(* Logix 5000 AddOnInstructionDefinition export Banner_R90C_R95C_R130C_Param_v4; software revision 33.00; part 2 of 3 *)
(* tags used below, declared in another part *)
   Hub : Banner_Hub_v4;
   Port_Data : Banner_IOL_Port_v4;
   Port : INT;
   Type : INT;   // 4 = R90C-4B21, 8 = R95C-8B21, 22 = R95-8B22
   Control : DINT;
   Command_Being_Processed : BOOL;
   Update_Archive : BOOL;
   Index_Write_Inprocess : INT;
   Index_Write_Control : INT;
   Inprocess_Index : DINT;
   Index1 : SINT;
   Index6 : SINT;
   Index5 : SINT;
(* Banner_R90C_R95C_R130C_Param_v4, continued *)

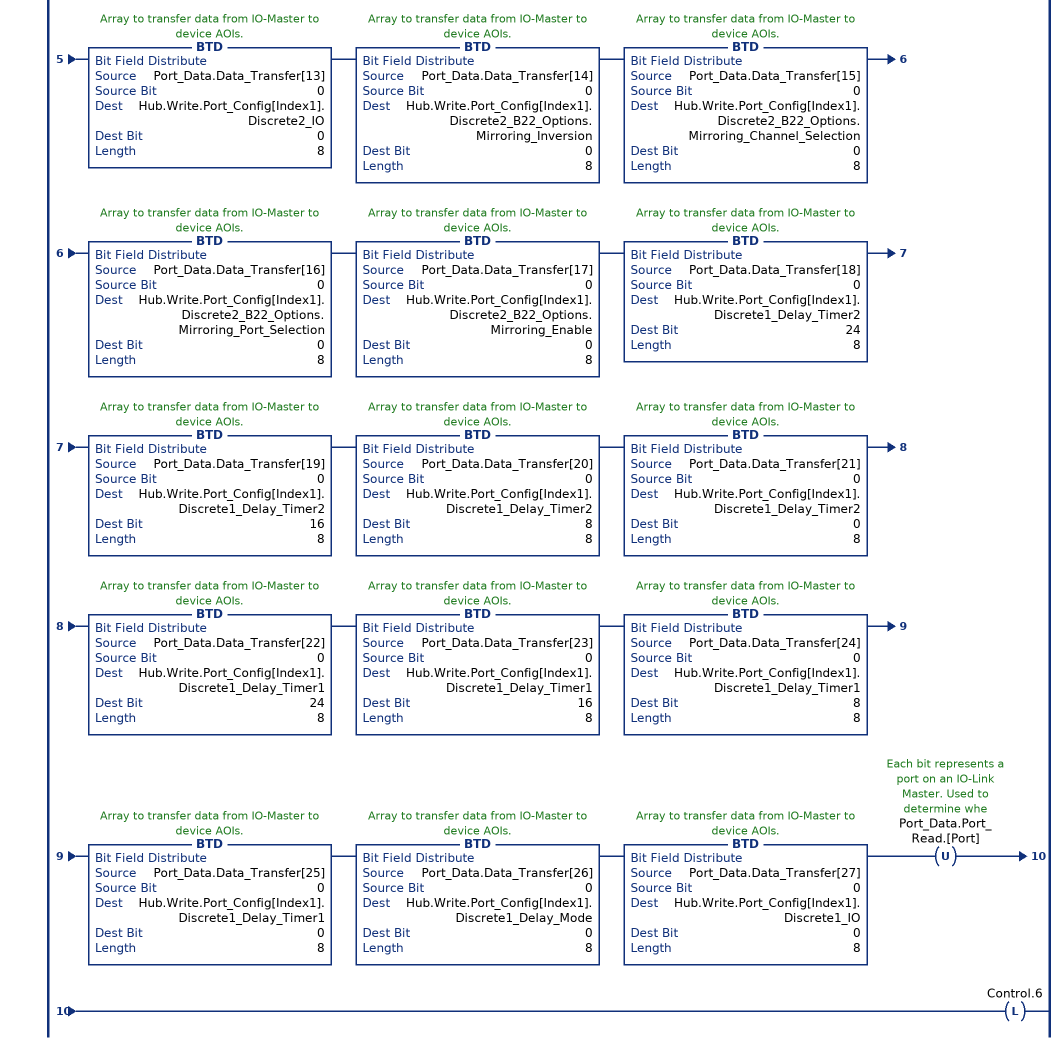
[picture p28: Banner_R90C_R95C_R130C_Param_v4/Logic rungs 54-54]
   54: XIC(Control.5)XIO(Control.6)GEQ(Hub.Command,13)LEQ(Hub.Command,20)EQU(Type,22)BTD(Port_Data.Data_Transfer[0],0,Hub.Write.Port_Config[Index1].Discrete2_B22_Options.Mirroring_Inversion,0,8)BTD(Port_Data.Data_Transfer[1],0,Hub.Write.Port_Config[Index1].Discrete2_B22_Options.Mirroring_Channel_Selection,0,8)BTD(Port_Data.Data_Transfer[2],0,Hub.Write.Port_Config[Index1].Discrete2_B22_Options.Mirroring_Port_Selection,0,8)BTD(Port_Data.Data_Transfer[3],0,Hub.Write.Port_Config[Index1].Discrete2_B22_Options.Mirroring_Enable,0,8)BTD(Port_Data.Data_Transfer[4],0,Hub.Write.Port_Config[Index1].Discrete2_Delay_Timer2,24,8)BTD(Port_Data.Data_Transfer[5],0,Hub.Write.Port_Config[Index1].Discrete2_Delay_Timer2,16,8)BTD(Port_Data.Data_Transfer[6],0,Hub.Write.Port_Config[Index1].Discrete2_Delay_Timer2,8,8)BTD(Port_Data.Data_Transfer[7],0,Hub.Write.Port_Config[Index1].Discrete2_Delay_Timer2,0,8)BTD(Port_Data.Data_Transfer[8],0,Hub.Write.Port_Config[Index1].Discrete2_Delay_Timer1,24,8)BTD(Port_Data.Data_Transfer[9],0,Hub.Write.Port_Config[Index1].Discrete2_Delay_Timer1,16,8)BTD(Port_Data.Data_Transfer[10],0,Hub.Write.Port_Config[Index1].Discrete2_Delay_Timer1,8,8)BTD(Port_Data.Data_Transfer[11],0,Hub.Write.Port_Config[Index1].Discrete2_Delay_Timer1,0,8)BTD(Port_Data.Data_Transfer[12],0,Hub.Write.Port_Config[Index1].Discrete2_Delay_Mode,0,8)BTD(Port_Data.Data_Transfer[13],0,Hub.Write.Port_Config[Index1].Discrete2_IO,0,8)BTD(Port_Data.Data_Transfer[14],0,Hub.Write.Port_Config[Index1].Discrete2_B22_Options.Mirroring_Inversion,0,8)BTD(Port_Data.Data_Transfer[15],0,Hub.Write.Port_Config[Index1].Discrete2_B22_Options.Mirroring_Channel_Selection,0,8)BTD(Port_Data.Data_Transfer[16],0,Hub.Write.Port_Config[Index1].Discrete2_B22_Options.Mirroring_Port_Selection,0,8)BTD(Port_Data.Data_Transfer[17],0,Hub.Write.Port_Config[Index1].Discrete2_B22_Options.Mirroring_Enable,0,8)BTD(Port_Data.Data_Transfer[18],0,Hub.Write.Port_Config[Index1].Discrete1_Delay_Timer2,24,8)BTD(Port_Data.Data_Transfer[19],0,Hub.Write.Port_Config[Index1].Discrete1_Delay_Timer2,16,8)BTD(Port_Data.Data_Transfer[20],0,Hub.Write.Port_Config[Index1].Discrete1_Delay_Timer2,8,8)BTD(Port_Data.Data_Transfer[21],0,Hub.Write.Port_Config[Index1].Discrete1_Delay_Timer2,0,8)BTD(Port_Data.Data_Transfer[22],0,Hub.Write.Port_Config[Index1].Discrete1_Delay_Timer1,24,8)BTD(Port_Data.Data_Transfer[23],0,Hub.Write.Port_Config[Index1].Discrete1_Delay_Timer1,16,8)BTD(Port_Data.Data_Transfer[24],0,Hub.Write.Port_Config[Index1].Discrete1_Delay_Timer1,8,8)BTD(Port_Data.Data_Transfer[25],0,Hub.Write.Port_Config[Index1].Discrete1_Delay_Timer1,0,8)BTD(Port_Data.Data_Transfer[26],0,Hub.Write.Port_Config[Index1].Discrete1_Delay_Mode,0,8)BTD(Port_Data.Data_Transfer[27],0,Hub.Write.Port_Config[Index1].Discrete1_IO,0,8)OTU(Port_Data.Port_Read.[Port])OTL(Control.6);
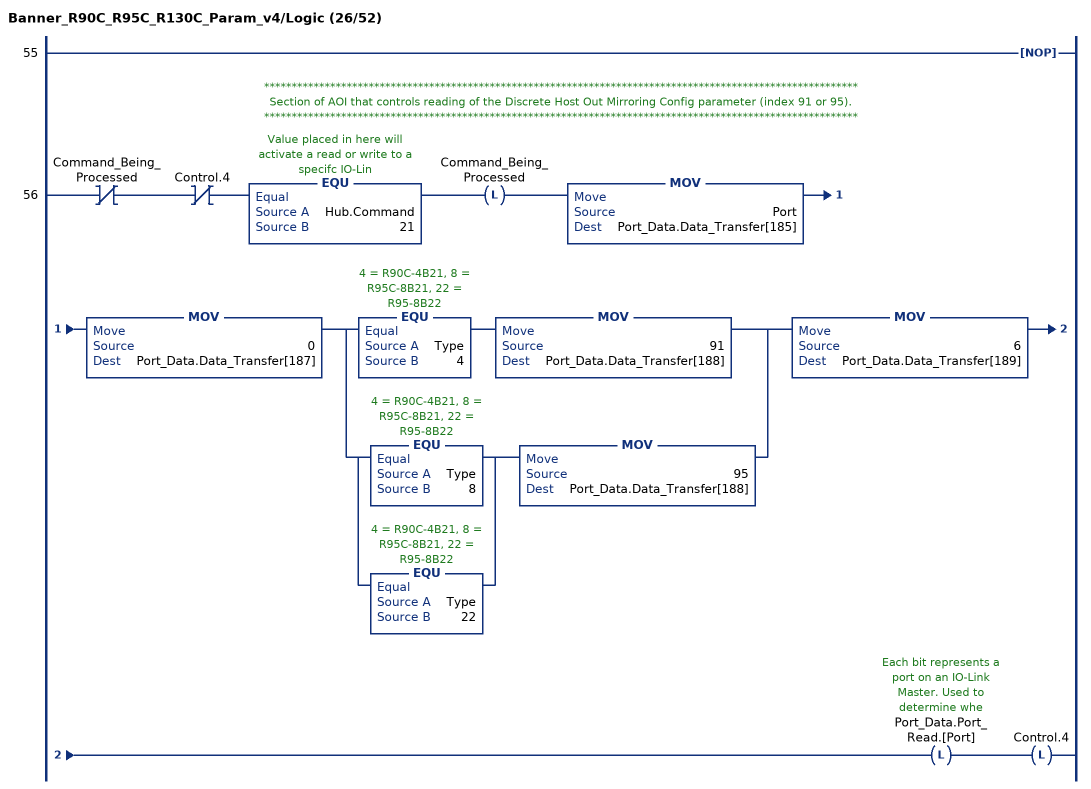
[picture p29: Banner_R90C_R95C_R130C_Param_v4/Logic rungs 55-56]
   55: NOP();
   // ************************************************************************************************************
   // Section of AOI that controls reading of the Discrete Host Out Mirroring Config parameter (index 91 or 95).
   // ************************************************************************************************************
   56: XIO(Command_Being_Processed)XIO(Control.4)EQU(Hub.Command,21)OTL(Command_Being_Processed)MOV(Port,Port_Data.Data_Transfer[185])MOV(0,Port_Data.Data_Transfer[187])[EQU(Type,4) MOV(91,Port_Data.Data_Transfer[188]) ,[EQU(Type,8) ,EQU(Type,22) ] MOV(95,Port_Data.Data_Transfer[188]) ]MOV(6,Port_Data.Data_Transfer[189])OTL(Port_Data.Port_Read.[Port])OTL(Control.4);
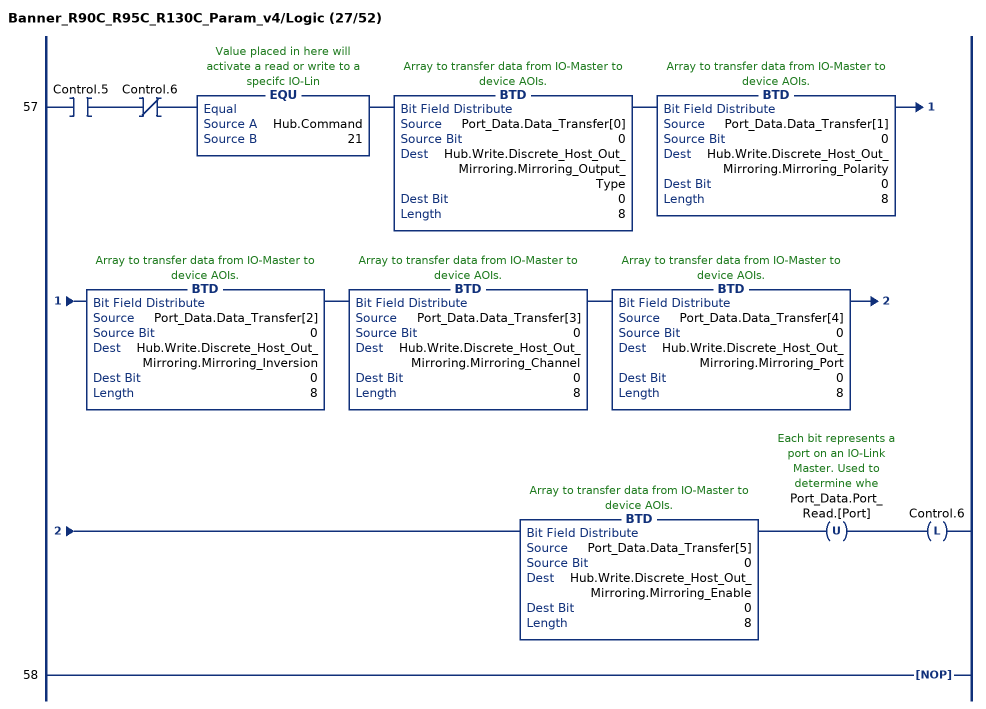
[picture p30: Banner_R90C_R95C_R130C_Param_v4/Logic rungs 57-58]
   57: XIC(Control.5)XIO(Control.6)EQU(Hub.Command,21)BTD(Port_Data.Data_Transfer[0],0,Hub.Write.Discrete_Host_Out_Mirroring.Mirroring_Output_Type,0,8)BTD(Port_Data.Data_Transfer[1],0,Hub.Write.Discrete_Host_Out_Mirroring.Mirroring_Polarity,0,8)BTD(Port_Data.Data_Transfer[2],0,Hub.Write.Discrete_Host_Out_Mirroring.Mirroring_Inversion,0,8)BTD(Port_Data.Data_Transfer[3],0,Hub.Write.Discrete_Host_Out_Mirroring.Mirroring_Channel,0,8)BTD(Port_Data.Data_Transfer[4],0,Hub.Write.Discrete_Host_Out_Mirroring.Mirroring_Port,0,8)BTD(Port_Data.Data_Transfer[5],0,Hub.Write.Discrete_Host_Out_Mirroring.Mirroring_Enable,0,8)OTU(Port_Data.Port_Read.[Port])OTL(Control.6);
   58: NOP();
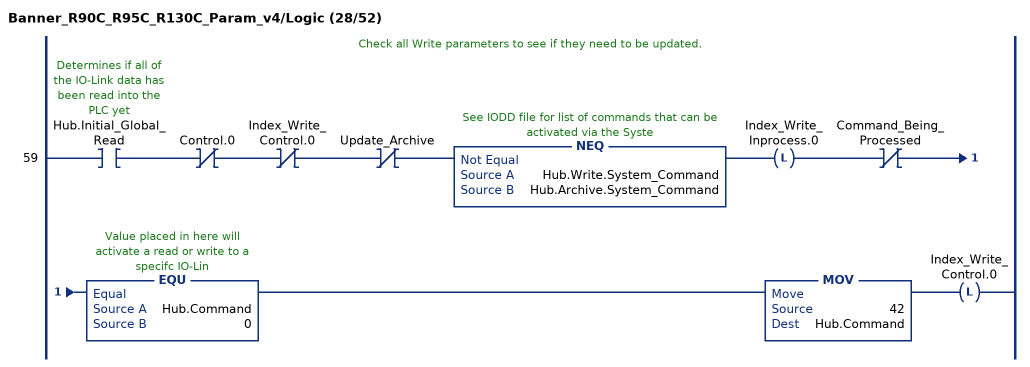
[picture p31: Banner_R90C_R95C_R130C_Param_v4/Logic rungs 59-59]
   // Check all Write parameters to see if they need to be updated.
   59: XIC(Hub.Initial_Global_Read)XIO(Control.0)XIO(Index_Write_Control.0)XIO(Update_Archive)NEQ(Hub.Write.System_Command,Hub.Archive.System_Command)OTL(Index_Write_Inprocess.0)XIO(Command_Being_Processed)EQU(Hub.Command,0)MOV(42,Hub.Command)OTL(Index_Write_Control.0);
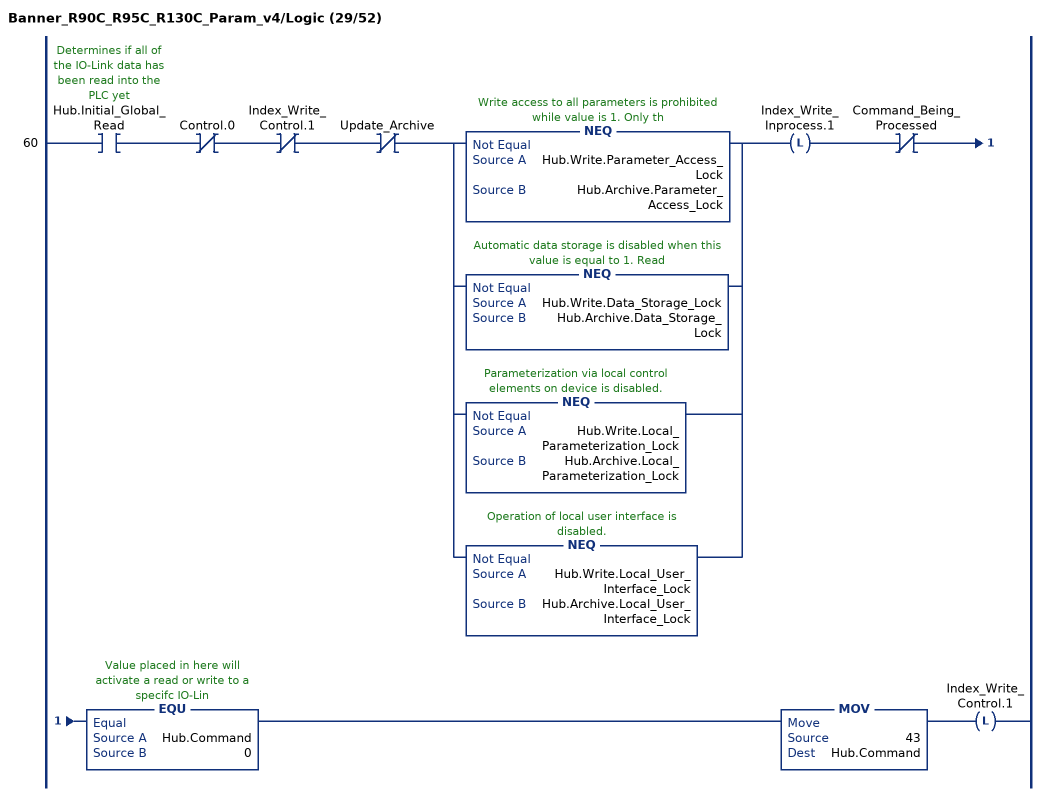
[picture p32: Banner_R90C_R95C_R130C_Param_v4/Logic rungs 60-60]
   60: XIC(Hub.Initial_Global_Read)XIO(Control.0)XIO(Index_Write_Control.1)XIO(Update_Archive)[NEQ(Hub.Write.Parameter_Access_Lock,Hub.Archive.Parameter_Access_Lock) ,NEQ(Hub.Write.Data_Storage_Lock,Hub.Archive.Data_Storage_Lock) ,NEQ(Hub.Write.Local_Parameterization_Lock,Hub.Archive.Local_Parameterization_Lock) ,NEQ(Hub.Write.Local_User_Interface_Lock,Hub.Archive.Local_User_Interface_Lock) ]OTL(Index_Write_Inprocess.1)XIO(Command_Being_Processed)EQU(Hub.Command,0)MOV(43,Hub.Command)OTL(Index_Write_Control.1);
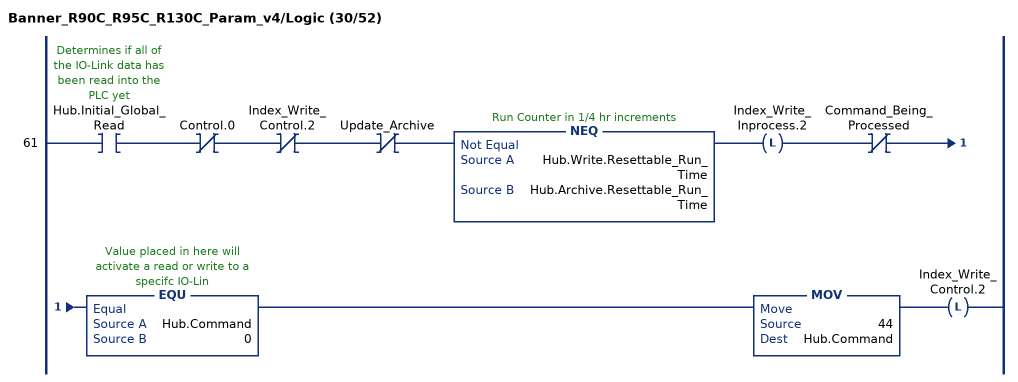
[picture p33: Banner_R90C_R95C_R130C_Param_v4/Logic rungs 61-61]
   61: XIC(Hub.Initial_Global_Read)XIO(Control.0)XIO(Index_Write_Control.2)XIO(Update_Archive)NEQ(Hub.Write.Resettable_Run_Time,Hub.Archive.Resettable_Run_Time)OTL(Index_Write_Inprocess.2)XIO(Command_Being_Processed)EQU(Hub.Command,0)MOV(44,Hub.Command)OTL(Index_Write_Control.2);
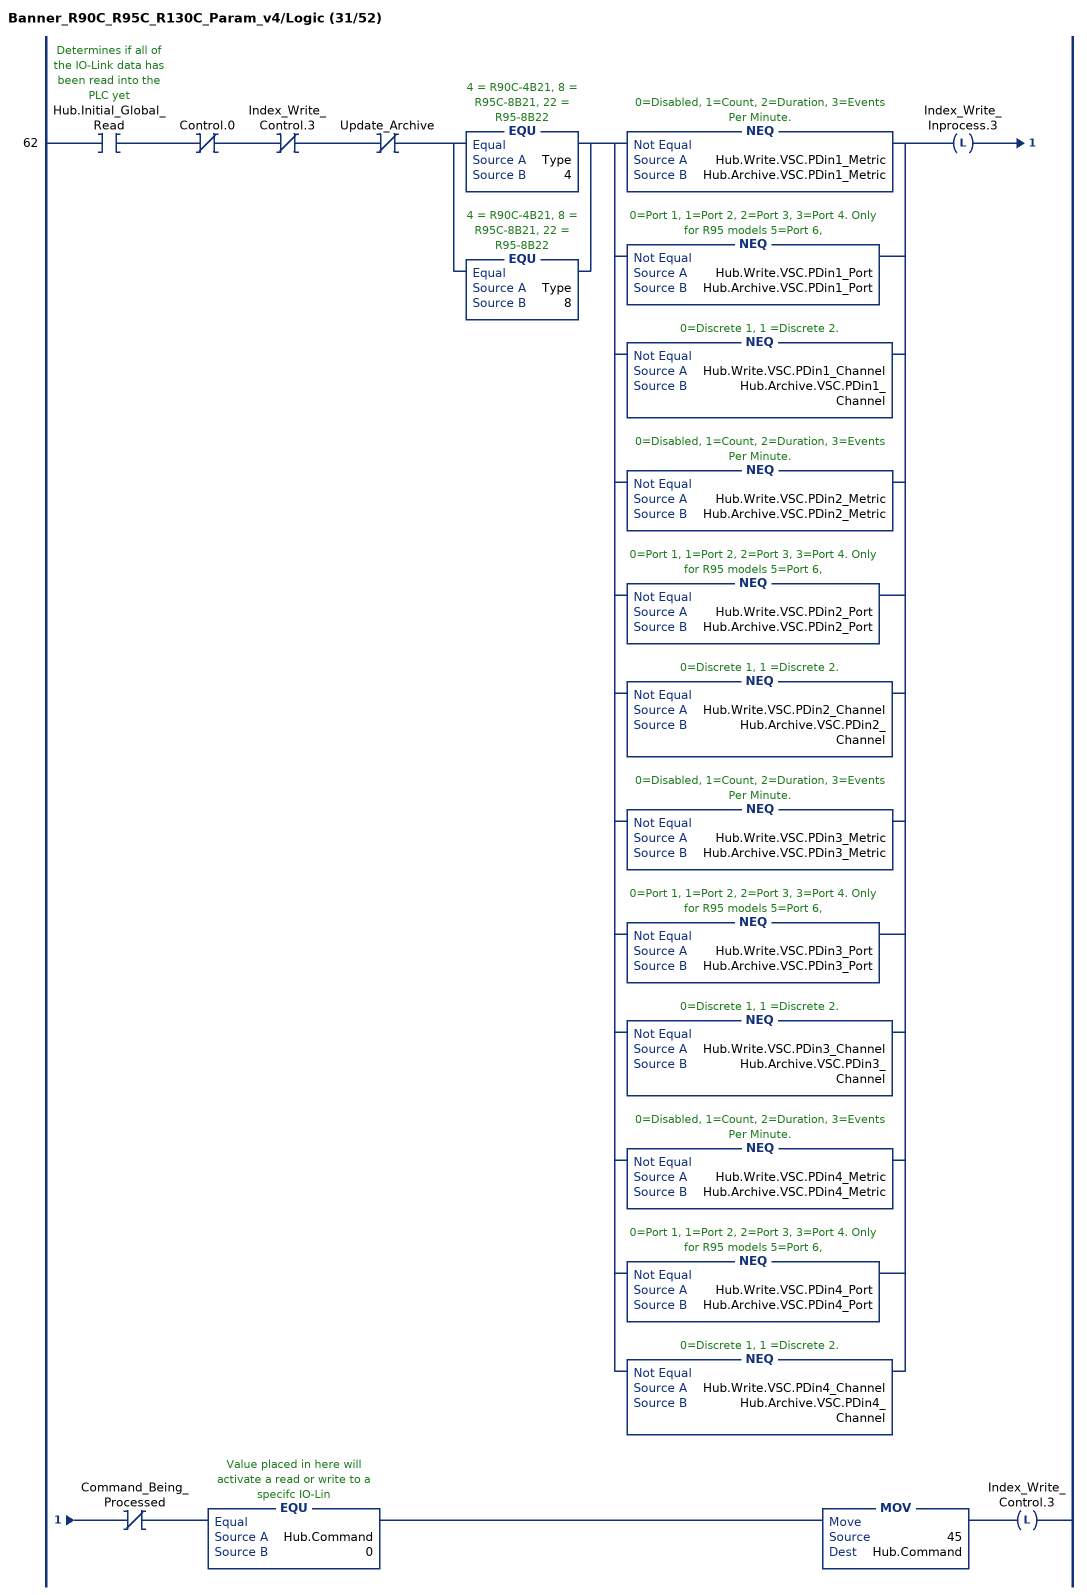
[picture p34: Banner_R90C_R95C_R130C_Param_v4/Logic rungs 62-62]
   62: XIC(Hub.Initial_Global_Read)XIO(Control.0)XIO(Index_Write_Control.3)XIO(Update_Archive)[EQU(Type,4) ,EQU(Type,8) ][NEQ(Hub.Write.VSC.PDin1_Metric,Hub.Archive.VSC.PDin1_Metric) ,NEQ(Hub.Write.VSC.PDin1_Port,Hub.Archive.VSC.PDin1_Port) ,NEQ(Hub.Write.VSC.PDin1_Channel,Hub.Archive.VSC.PDin1_Channel) ,NEQ(Hub.Write.VSC.PDin2_Metric,Hub.Archive.VSC.PDin2_Metric) ,NEQ(Hub.Write.VSC.PDin2_Port,Hub.Archive.VSC.PDin2_Port) ,NEQ(Hub.Write.VSC.PDin2_Channel,Hub.Archive.VSC.PDin2_Channel) ,NEQ(Hub.Write.VSC.PDin3_Metric,Hub.Archive.VSC.PDin3_Metric) ,NEQ(Hub.Write.VSC.PDin3_Port,Hub.Archive.VSC.PDin3_Port) ,NEQ(Hub.Write.VSC.PDin3_Channel,Hub.Archive.VSC.PDin3_Channel) ,NEQ(Hub.Write.VSC.PDin4_Metric,Hub.Archive.VSC.PDin4_Metric) ,NEQ(Hub.Write.VSC.PDin4_Port,Hub.Archive.VSC.PDin4_Port) ,NEQ(Hub.Write.VSC.PDin4_Channel,Hub.Archive.VSC.PDin4_Channel) ]OTL(Index_Write_Inprocess.3)XIO(Command_Being_Processed)EQU(Hub.Command,0)MOV(45,Hub.Command)OTL(Index_Write_Control.3);
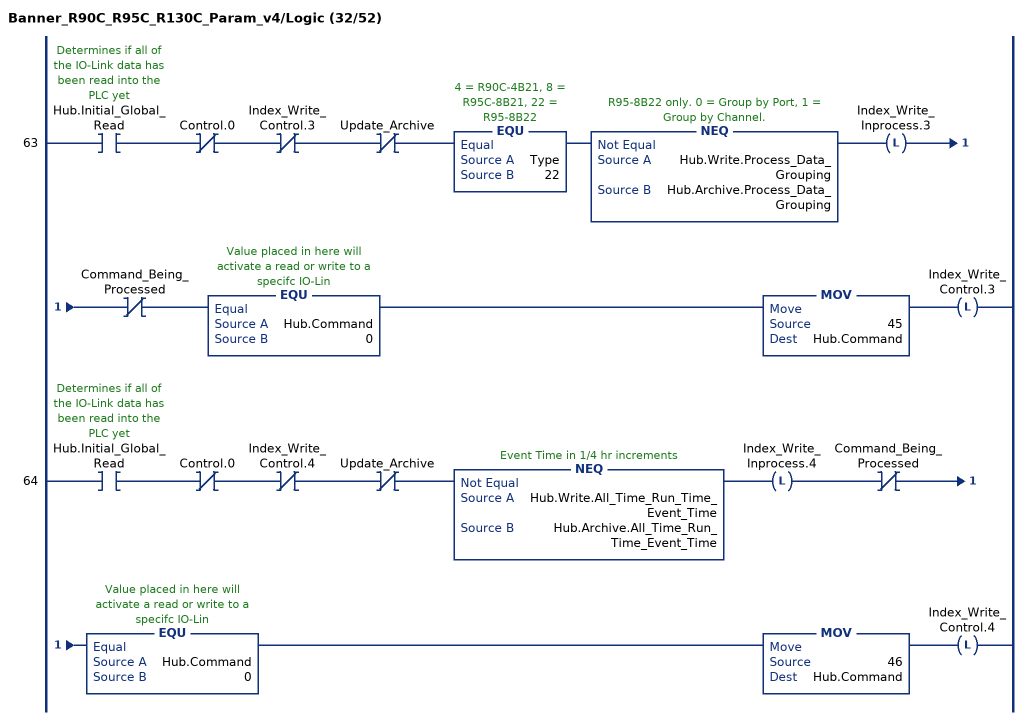
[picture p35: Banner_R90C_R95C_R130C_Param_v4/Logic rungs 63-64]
   63: XIC(Hub.Initial_Global_Read)XIO(Control.0)XIO(Index_Write_Control.3)XIO(Update_Archive)EQU(Type,22)NEQ(Hub.Write.Process_Data_Grouping,Hub.Archive.Process_Data_Grouping)OTL(Index_Write_Inprocess.3)XIO(Command_Being_Processed)EQU(Hub.Command,0)MOV(45,Hub.Command)OTL(Index_Write_Control.3);
   64: XIC(Hub.Initial_Global_Read)XIO(Control.0)XIO(Index_Write_Control.4)XIO(Update_Archive)NEQ(Hub.Write.All_Time_Run_Time_Event_Time,Hub.Archive.All_Time_Run_Time_Event_Time)OTL(Index_Write_Inprocess.4)XIO(Command_Being_Processed)EQU(Hub.Command,0)MOV(46,Hub.Command)OTL(Index_Write_Control.4);
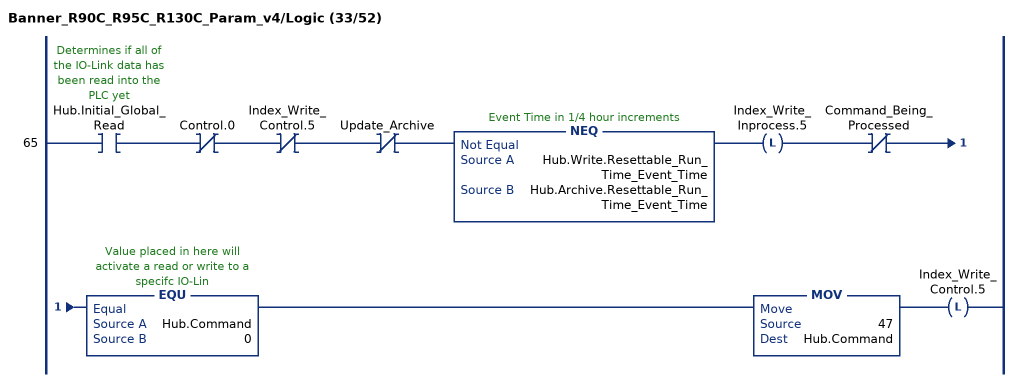
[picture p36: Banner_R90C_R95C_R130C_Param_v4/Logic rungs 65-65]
   65: XIC(Hub.Initial_Global_Read)XIO(Control.0)XIO(Index_Write_Control.5)XIO(Update_Archive)NEQ(Hub.Write.Resettable_Run_Time_Event_Time,Hub.Archive.Resettable_Run_Time_Event_Time)OTL(Index_Write_Inprocess.5)XIO(Command_Being_Processed)EQU(Hub.Command,0)MOV(47,Hub.Command)OTL(Index_Write_Control.5);
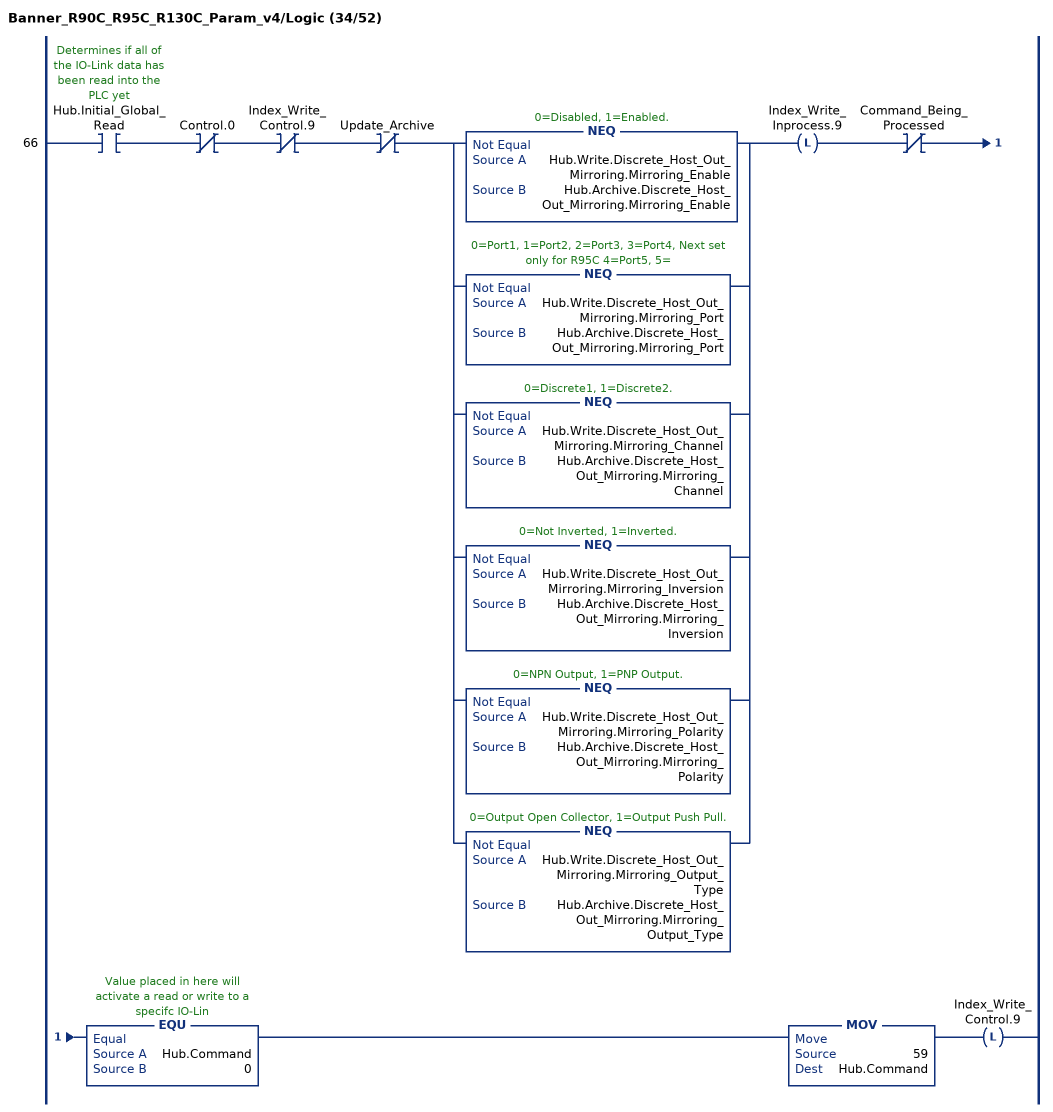
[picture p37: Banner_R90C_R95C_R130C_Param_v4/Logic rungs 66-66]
   66: XIC(Hub.Initial_Global_Read)XIO(Control.0)XIO(Index_Write_Control.9)XIO(Update_Archive)[NEQ(Hub.Write.Discrete_Host_Out_Mirroring.Mirroring_Enable,Hub.Archive.Discrete_Host_Out_Mirroring.Mirroring_Enable) ,NEQ(Hub.Write.Discrete_Host_Out_Mirroring.Mirroring_Port,Hub.Archive.Discrete_Host_Out_Mirroring.Mirroring_Port) ,NEQ(Hub.Write.Discrete_Host_Out_Mirroring.Mirroring_Channel,Hub.Archive.Discrete_Host_Out_Mirroring.Mirroring_Channel) ,NEQ(Hub.Write.Discrete_Host_Out_Mirroring.Mirroring_Inversion,Hub.Archive.Discrete_Host_Out_Mirroring.Mirroring_Inversion) ,NEQ(Hub.Write.Discrete_Host_Out_Mirroring.Mirroring_Polarity,Hub.Archive.Discrete_Host_Out_Mirroring.Mirroring_Polarity) ,NEQ(Hub.Write.Discrete_Host_Out_Mirroring.Mirroring_Output_Type,Hub.Archive.Discrete_Host_Out_Mirroring.Mirroring_Output_Type) ]OTL(Index_Write_Inprocess.9)XIO(Command_Being_Processed)EQU(Hub.Command,0)MOV(59,Hub.Command)OTL(Index_Write_Control.9);
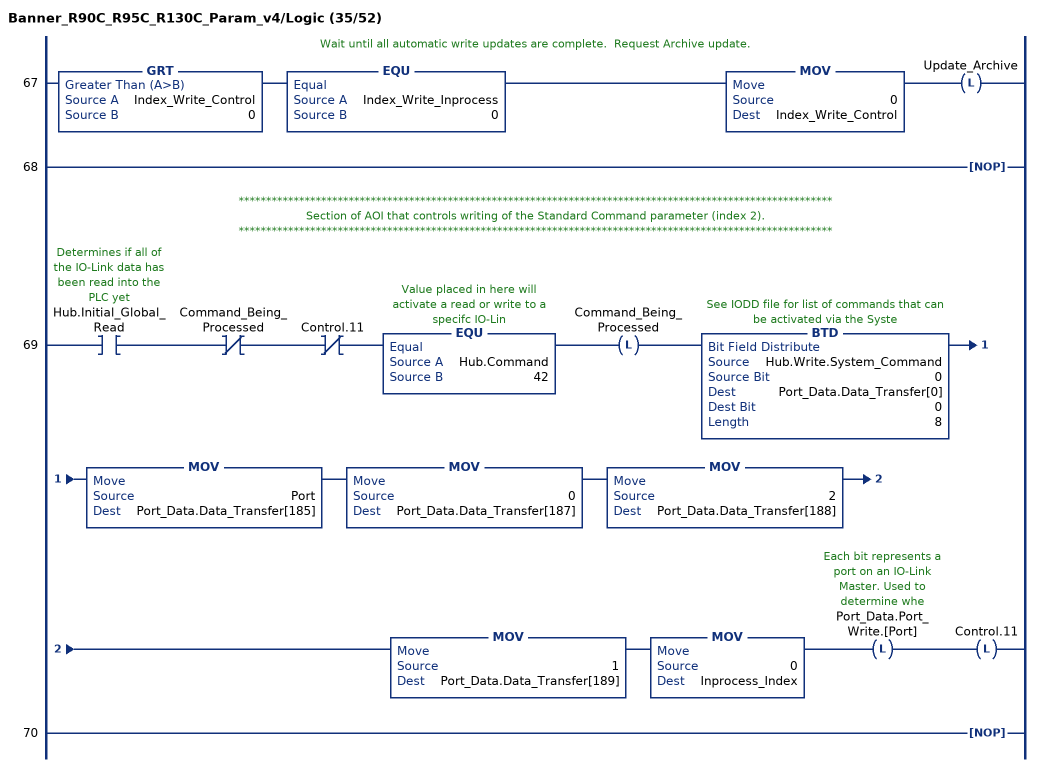
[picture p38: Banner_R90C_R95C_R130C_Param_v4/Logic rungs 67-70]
   // Wait until all automatic write updates are complete.  Request Archive update.
   67: GRT(Index_Write_Control,0)EQU(Index_Write_Inprocess,0)MOV(0,Index_Write_Control)OTL(Update_Archive);
   68: NOP();
   // ************************************************************************************************************
   // Section of AOI that controls writing of the Standard Command parameter (index 2).
   // ************************************************************************************************************
   69: XIC(Hub.Initial_Global_Read)XIO(Command_Being_Processed)XIO(Control.11)EQU(Hub.Command,42)OTL(Command_Being_Processed)BTD(Hub.Write.System_Command,0,Port_Data.Data_Transfer[0],0,8)MOV(Port,Port_Data.Data_Transfer[185])MOV(0,Port_Data.Data_Transfer[187])MOV(2,Port_Data.Data_Transfer[188])MOV(1,Port_Data.Data_Transfer[189])MOV(0,Inprocess_Index)OTL(Port_Data.Port_Write.[Port])OTL(Control.11);
   70: NOP();
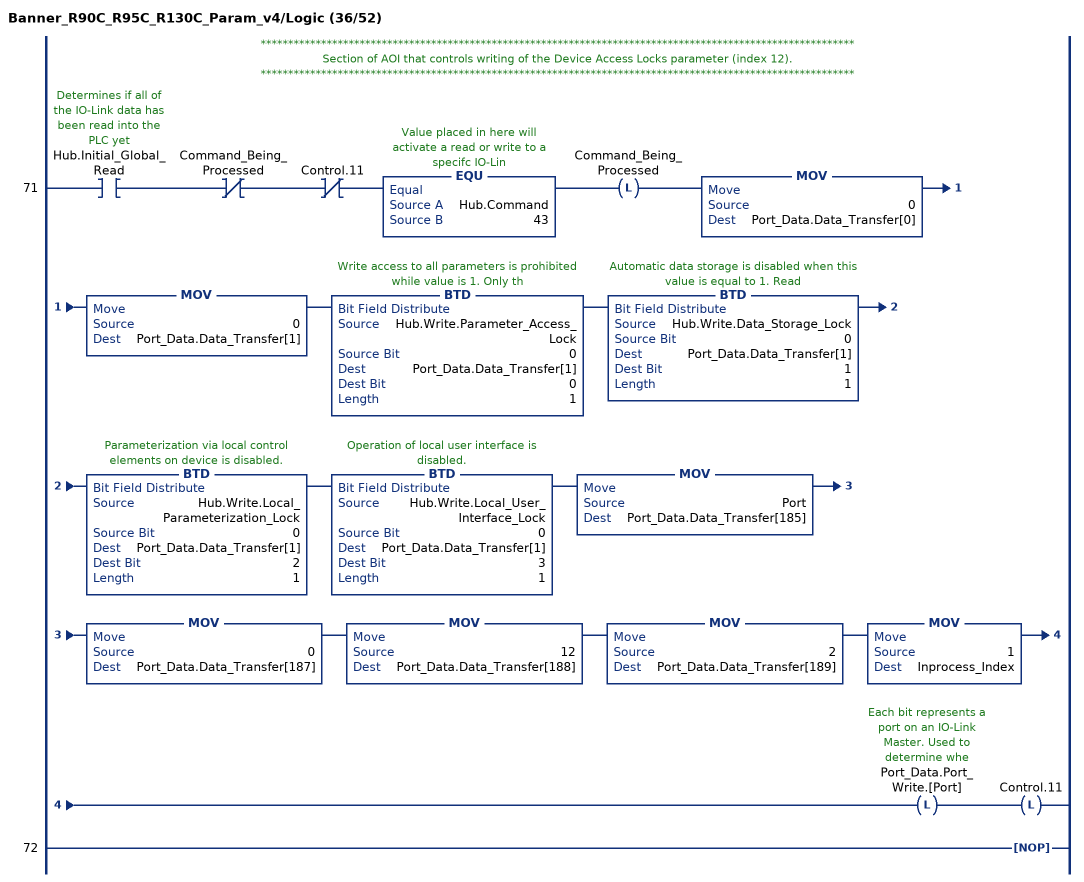
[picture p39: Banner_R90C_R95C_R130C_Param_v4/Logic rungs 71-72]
   // ************************************************************************************************************
   // Section of AOI that controls writing of the Device Access Locks parameter (index 12).
   // ************************************************************************************************************
   71: XIC(Hub.Initial_Global_Read)XIO(Command_Being_Processed)XIO(Control.11)EQU(Hub.Command,43)OTL(Command_Being_Processed)MOV(0,Port_Data.Data_Transfer[0])MOV(0,Port_Data.Data_Transfer[1])BTD(Hub.Write.Parameter_Access_Lock,0,Port_Data.Data_Transfer[1],0,1)BTD(Hub.Write.Data_Storage_Lock,0,Port_Data.Data_Transfer[1],1,1)BTD(Hub.Write.Local_Parameterization_Lock,0,Port_Data.Data_Transfer[1],2,1)BTD(Hub.Write.Local_User_Interface_Lock,0,Port_Data.Data_Transfer[1],3,1)MOV(Port,Port_Data.Data_Transfer[185])MOV(0,Port_Data.Data_Transfer[187])MOV(12,Port_Data.Data_Transfer[188])MOV(2,Port_Data.Data_Transfer[189])MOV(1,Inprocess_Index)OTL(Port_Data.Port_Write.[Port])OTL(Control.11);
   72: NOP();
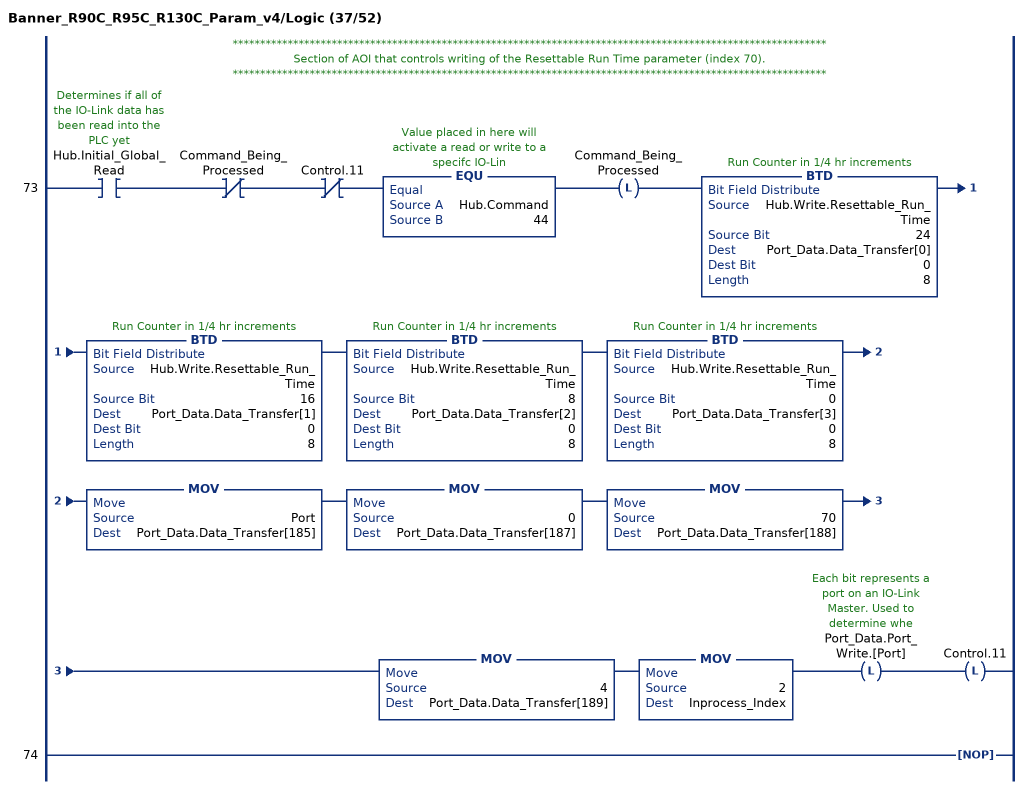
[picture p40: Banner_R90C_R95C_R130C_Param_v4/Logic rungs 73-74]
   // ************************************************************************************************************
   // Section of AOI that controls writing of the Resettable Run Time parameter (index 70).
   // ************************************************************************************************************
   73: XIC(Hub.Initial_Global_Read)XIO(Command_Being_Processed)XIO(Control.11)EQU(Hub.Command,44)OTL(Command_Being_Processed)BTD(Hub.Write.Resettable_Run_Time,24,Port_Data.Data_Transfer[0],0,8)BTD(Hub.Write.Resettable_Run_Time,16,Port_Data.Data_Transfer[1],0,8)BTD(Hub.Write.Resettable_Run_Time,8,Port_Data.Data_Transfer[2],0,8)BTD(Hub.Write.Resettable_Run_Time,0,Port_Data.Data_Transfer[3],0,8)MOV(Port,Port_Data.Data_Transfer[185])MOV(0,Port_Data.Data_Transfer[187])MOV(70,Port_Data.Data_Transfer[188])MOV(4,Port_Data.Data_Transfer[189])MOV(2,Inprocess_Index)OTL(Port_Data.Port_Write.[Port])OTL(Control.11);
   74: NOP();
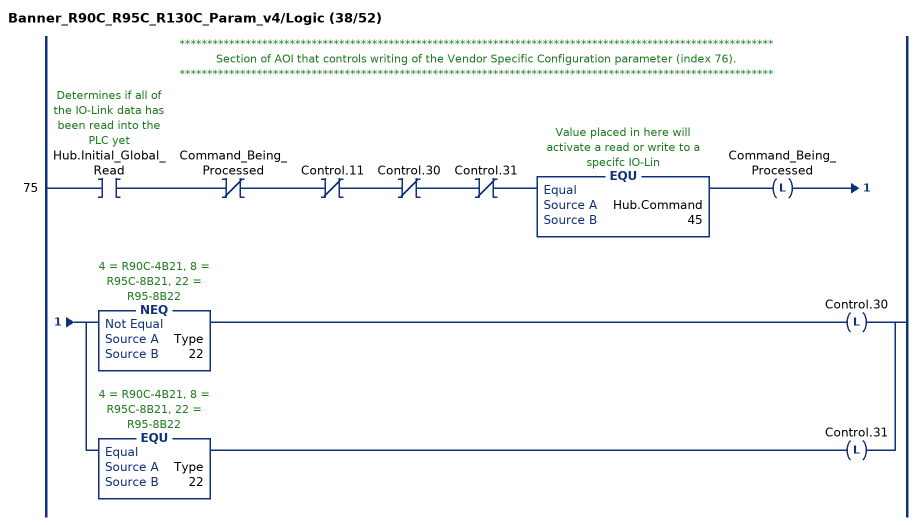
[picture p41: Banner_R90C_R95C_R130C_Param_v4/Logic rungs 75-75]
   // ************************************************************************************************************
   // Section of AOI that controls writing of the Vendor Specific Configuration parameter (index 76).
   // ************************************************************************************************************
   75: XIC(Hub.Initial_Global_Read)XIO(Command_Being_Processed)XIO(Control.11)XIO(Control.30)XIO(Control.31)EQU(Hub.Command,45)OTL(Command_Being_Processed)[NEQ(Type,22) OTL(Control.30) ,EQU(Type,22) OTL(Control.31) ];
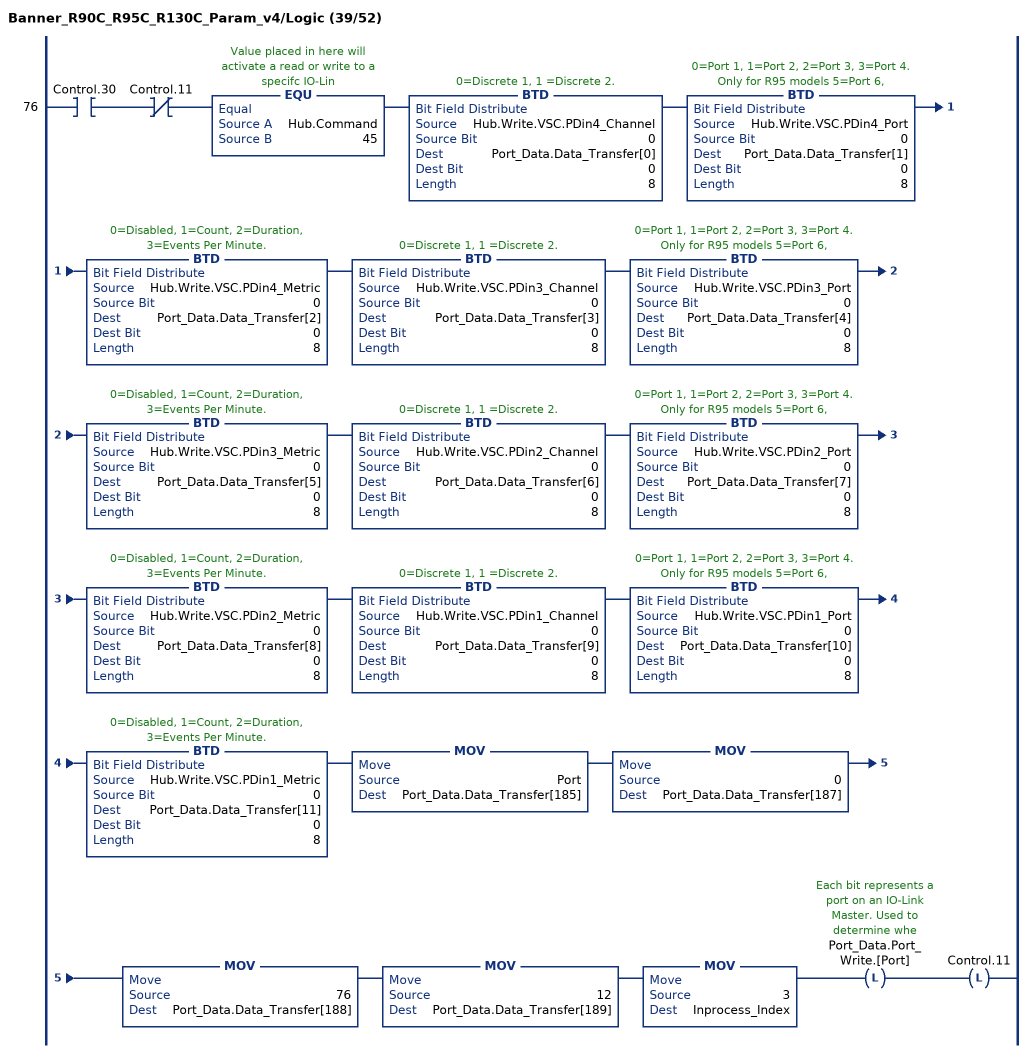
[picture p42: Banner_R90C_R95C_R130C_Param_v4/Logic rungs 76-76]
   76: XIC(Control.30)XIO(Control.11)EQU(Hub.Command,45)BTD(Hub.Write.VSC.PDin4_Channel,0,Port_Data.Data_Transfer[0],0,8)BTD(Hub.Write.VSC.PDin4_Port,0,Port_Data.Data_Transfer[1],0,8)BTD(Hub.Write.VSC.PDin4_Metric,0,Port_Data.Data_Transfer[2],0,8)BTD(Hub.Write.VSC.PDin3_Channel,0,Port_Data.Data_Transfer[3],0,8)BTD(Hub.Write.VSC.PDin3_Port,0,Port_Data.Data_Transfer[4],0,8)BTD(Hub.Write.VSC.PDin3_Metric,0,Port_Data.Data_Transfer[5],0,8)BTD(Hub.Write.VSC.PDin2_Channel,0,Port_Data.Data_Transfer[6],0,8)BTD(Hub.Write.VSC.PDin2_Port,0,Port_Data.Data_Transfer[7],0,8)BTD(Hub.Write.VSC.PDin2_Metric,0,Port_Data.Data_Transfer[8],0,8)BTD(Hub.Write.VSC.PDin1_Channel,0,Port_Data.Data_Transfer[9],0,8)BTD(Hub.Write.VSC.PDin1_Port,0,Port_Data.Data_Transfer[10],0,8)BTD(Hub.Write.VSC.PDin1_Metric,0,Port_Data.Data_Transfer[11],0,8)MOV(Port,Port_Data.Data_Transfer[185])MOV(0,Port_Data.Data_Transfer[187])MOV(76,Port_Data.Data_Transfer[188])MOV(12,Port_Data.Data_Transfer[189])MOV(3,Inprocess_Index)OTL(Port_Data.Port_Write.[Port])OTL(Control.11);
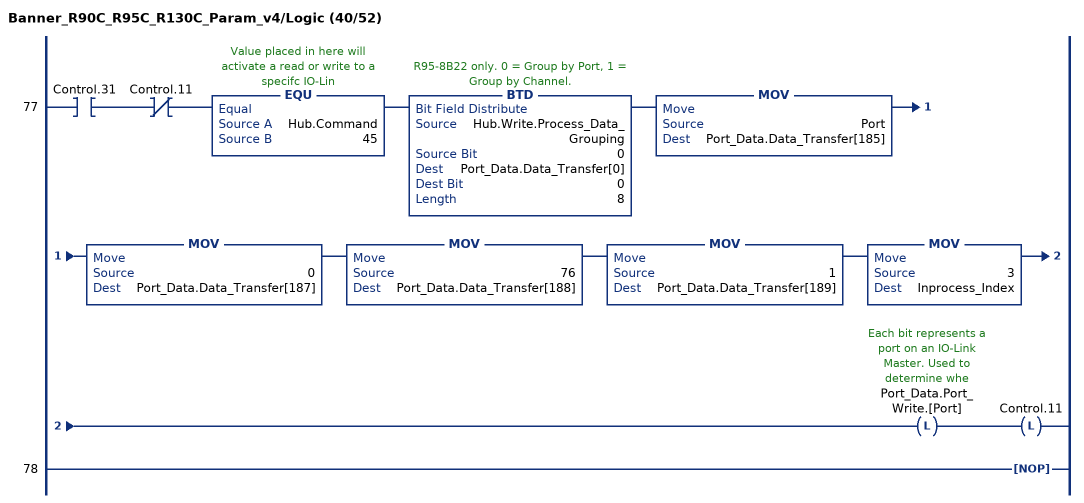
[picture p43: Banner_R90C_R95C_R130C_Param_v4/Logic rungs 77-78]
   77: XIC(Control.31)XIO(Control.11)EQU(Hub.Command,45)BTD(Hub.Write.Process_Data_Grouping,0,Port_Data.Data_Transfer[0],0,8)MOV(Port,Port_Data.Data_Transfer[185])MOV(0,Port_Data.Data_Transfer[187])MOV(76,Port_Data.Data_Transfer[188])MOV(1,Port_Data.Data_Transfer[189])MOV(3,Inprocess_Index)OTL(Port_Data.Port_Write.[Port])OTL(Control.11);
   78: NOP();
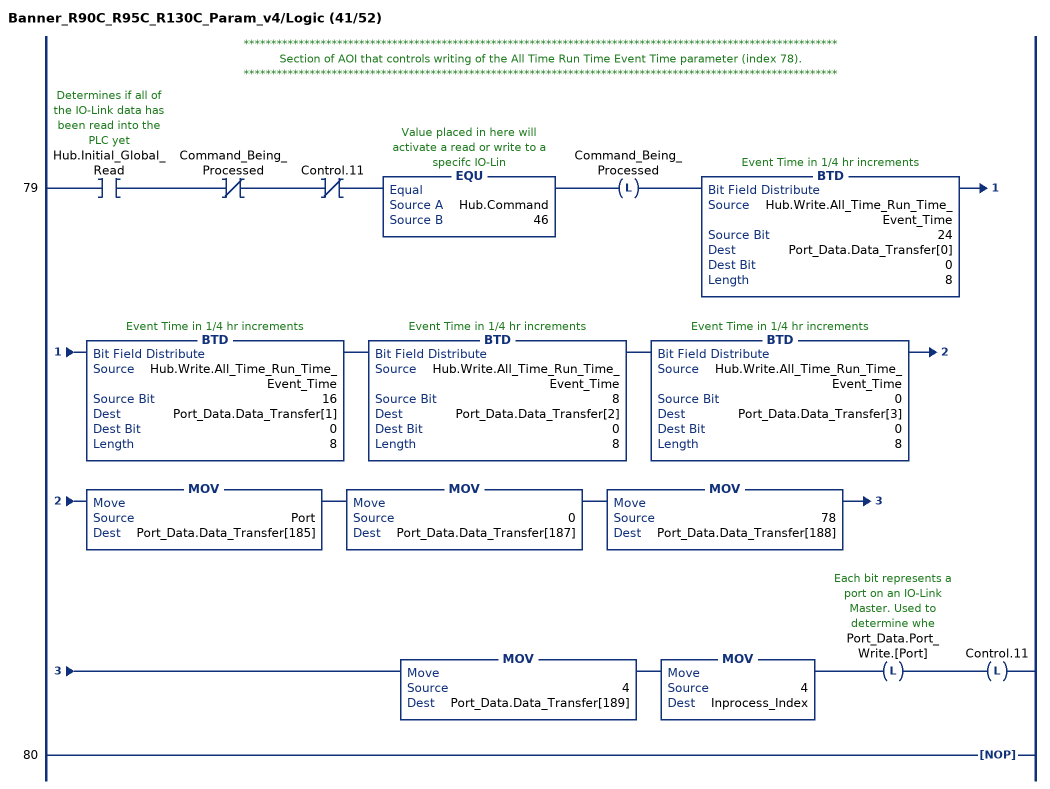
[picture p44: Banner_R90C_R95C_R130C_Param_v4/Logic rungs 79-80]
   // ************************************************************************************************************
   // Section of AOI that controls writing of the All Time Run Time Event Time parameter (index 78).
   // ************************************************************************************************************
   79: XIC(Hub.Initial_Global_Read)XIO(Command_Being_Processed)XIO(Control.11)EQU(Hub.Command,46)OTL(Command_Being_Processed)BTD(Hub.Write.All_Time_Run_Time_Event_Time,24,Port_Data.Data_Transfer[0],0,8)BTD(Hub.Write.All_Time_Run_Time_Event_Time,16,Port_Data.Data_Transfer[1],0,8)BTD(Hub.Write.All_Time_Run_Time_Event_Time,8,Port_Data.Data_Transfer[2],0,8)BTD(Hub.Write.All_Time_Run_Time_Event_Time,0,Port_Data.Data_Transfer[3],0,8)MOV(Port,Port_Data.Data_Transfer[185])MOV(0,Port_Data.Data_Transfer[187])MOV(78,Port_Data.Data_Transfer[188])MOV(4,Port_Data.Data_Transfer[189])MOV(4,Inprocess_Index)OTL(Port_Data.Port_Write.[Port])OTL(Control.11);
   80: NOP();
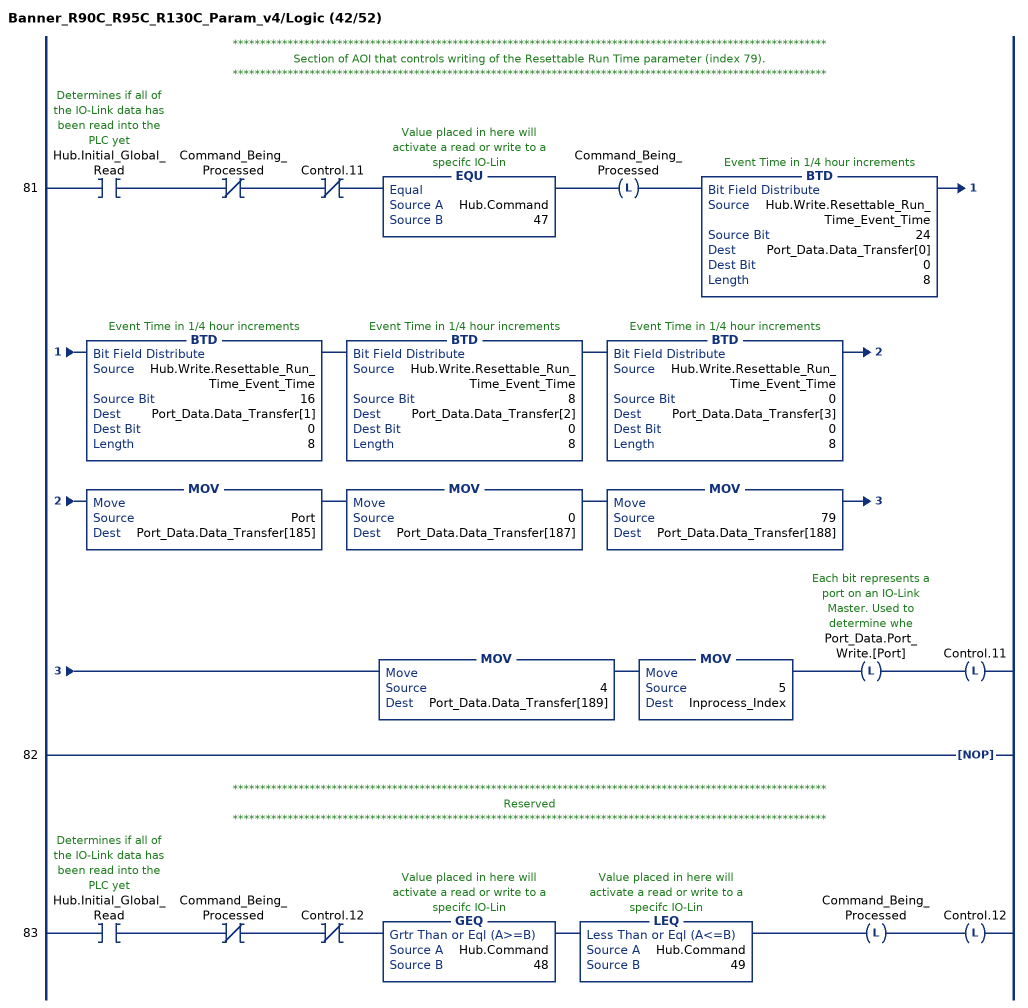
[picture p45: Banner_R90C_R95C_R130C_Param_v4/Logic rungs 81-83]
   // ************************************************************************************************************
   // Section of AOI that controls writing of the Resettable Run Time parameter (index 79).
   // ************************************************************************************************************
   81: XIC(Hub.Initial_Global_Read)XIO(Command_Being_Processed)XIO(Control.11)EQU(Hub.Command,47)OTL(Command_Being_Processed)BTD(Hub.Write.Resettable_Run_Time_Event_Time,24,Port_Data.Data_Transfer[0],0,8)BTD(Hub.Write.Resettable_Run_Time_Event_Time,16,Port_Data.Data_Transfer[1],0,8)BTD(Hub.Write.Resettable_Run_Time_Event_Time,8,Port_Data.Data_Transfer[2],0,8)BTD(Hub.Write.Resettable_Run_Time_Event_Time,0,Port_Data.Data_Transfer[3],0,8)MOV(Port,Port_Data.Data_Transfer[185])MOV(0,Port_Data.Data_Transfer[187])MOV(79,Port_Data.Data_Transfer[188])MOV(4,Port_Data.Data_Transfer[189])MOV(5,Inprocess_Index)OTL(Port_Data.Port_Write.[Port])OTL(Control.11);
   82: NOP();
   // ************************************************************************************************************
   // Reserved
   // ************************************************************************************************************
   83: XIC(Hub.Initial_Global_Read)XIO(Command_Being_Processed)XIO(Control.12)GEQ(Hub.Command,48)LEQ(Hub.Command,49)OTL(Command_Being_Processed)OTL(Control.12);
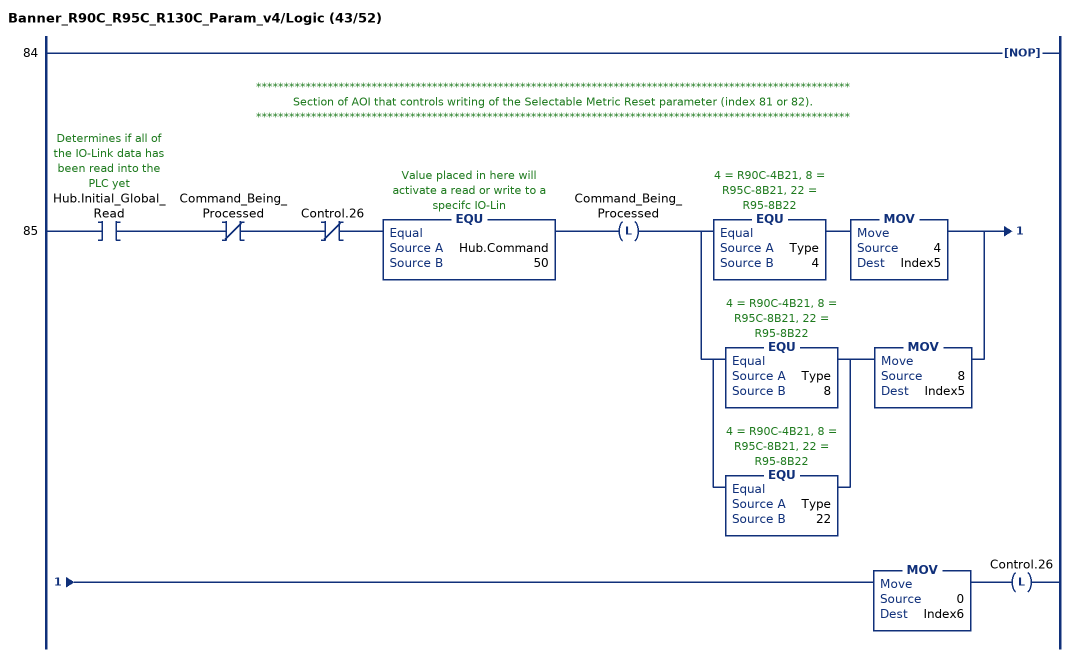
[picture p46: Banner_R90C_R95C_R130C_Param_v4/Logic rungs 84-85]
   84: NOP();
   // ************************************************************************************************************
   // Section of AOI that controls writing of the Selectable Metric Reset parameter (index 81 or 82).
   // ************************************************************************************************************
   85: XIC(Hub.Initial_Global_Read)XIO(Command_Being_Processed)XIO(Control.26)EQU(Hub.Command,50)OTL(Command_Being_Processed)[EQU(Type,4) MOV(4,Index5) ,[EQU(Type,8) ,EQU(Type,22) ] MOV(8,Index5) ]MOV(0,Index6)OTL(Control.26);
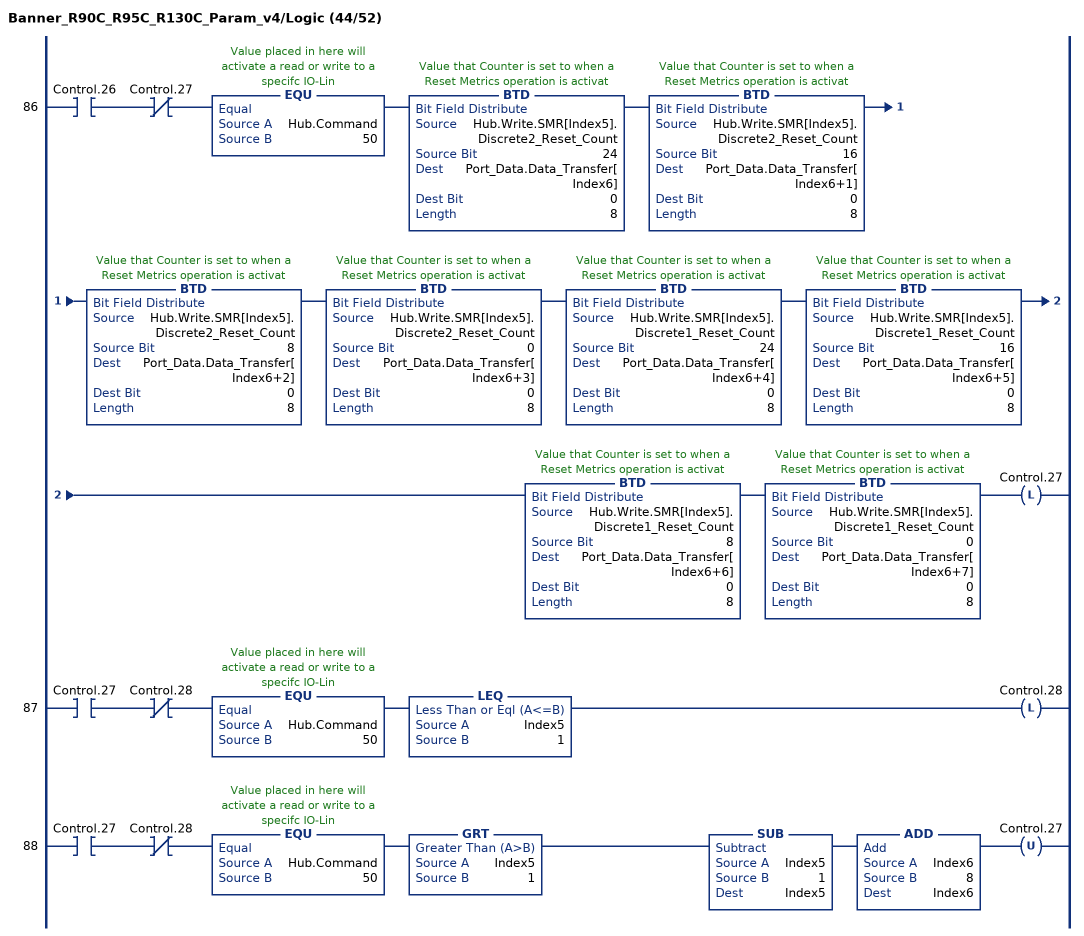
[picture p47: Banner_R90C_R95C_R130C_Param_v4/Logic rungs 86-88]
   86: XIC(Control.26)XIO(Control.27)EQU(Hub.Command,50)BTD(Hub.Write.SMR[Index5].Discrete2_Reset_Count,24,Port_Data.Data_Transfer[Index6],0,8)BTD(Hub.Write.SMR[Index5].Discrete2_Reset_Count,16,Port_Data.Data_Transfer[Index6+1],0,8)BTD(Hub.Write.SMR[Index5].Discrete2_Reset_Count,8,Port_Data.Data_Transfer[Index6+2],0,8)BTD(Hub.Write.SMR[Index5].Discrete2_Reset_Count,0,Port_Data.Data_Transfer[Index6+3],0,8)BTD(Hub.Write.SMR[Index5].Discrete1_Reset_Count,24,Port_Data.Data_Transfer[Index6+4],0,8)BTD(Hub.Write.SMR[Index5].Discrete1_Reset_Count,16,Port_Data.Data_Transfer[Index6+5],0,8)BTD(Hub.Write.SMR[Index5].Discrete1_Reset_Count,8,Port_Data.Data_Transfer[Index6+6],0,8)BTD(Hub.Write.SMR[Index5].Discrete1_Reset_Count,0,Port_Data.Data_Transfer[Index6+7],0,8)OTL(Control.27);
   87: XIC(Control.27)XIO(Control.28)EQU(Hub.Command,50)LEQ(Index5,1)OTL(Control.28);
   88: XIC(Control.27)XIO(Control.28)EQU(Hub.Command,50)GRT(Index5,1)SUB(Index5,1,Index5)ADD(Index6,8,Index6)OTU(Control.27);
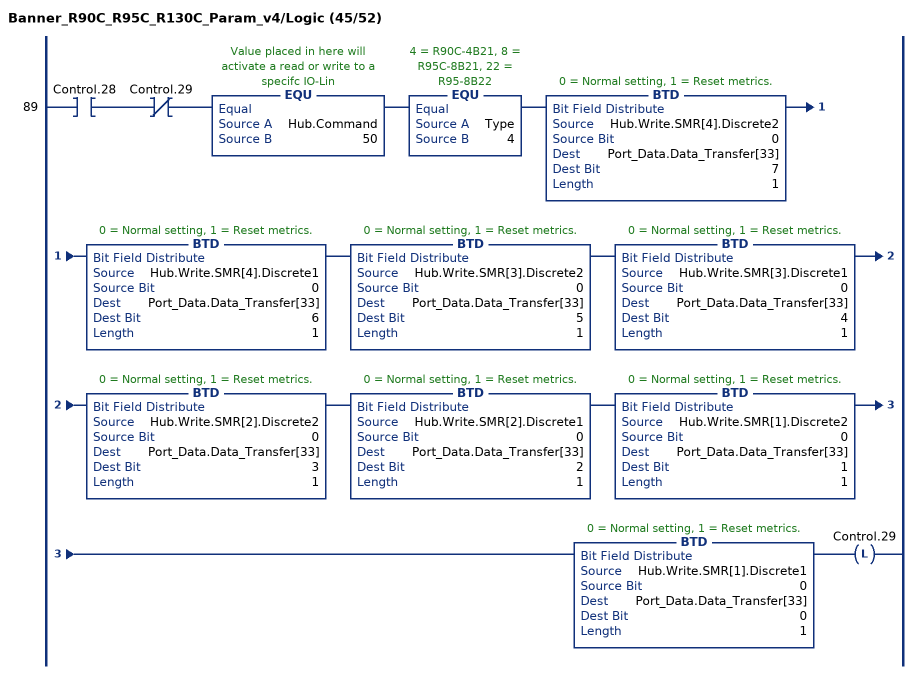
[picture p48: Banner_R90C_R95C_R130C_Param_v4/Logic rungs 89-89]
   89: XIC(Control.28)XIO(Control.29)EQU(Hub.Command,50)EQU(Type,4)BTD(Hub.Write.SMR[4].Discrete2,0,Port_Data.Data_Transfer[33],7,1)BTD(Hub.Write.SMR[4].Discrete1,0,Port_Data.Data_Transfer[33],6,1)BTD(Hub.Write.SMR[3].Discrete2,0,Port_Data.Data_Transfer[33],5,1)BTD(Hub.Write.SMR[3].Discrete1,0,Port_Data.Data_Transfer[33],4,1)BTD(Hub.Write.SMR[2].Discrete2,0,Port_Data.Data_Transfer[33],3,1)BTD(Hub.Write.SMR[2].Discrete1,0,Port_Data.Data_Transfer[33],2,1)BTD(Hub.Write.SMR[1].Discrete2,0,Port_Data.Data_Transfer[33],1,1)BTD(Hub.Write.SMR[1].Discrete1,0,Port_Data.Data_Transfer[33],0,1)OTL(Control.29);
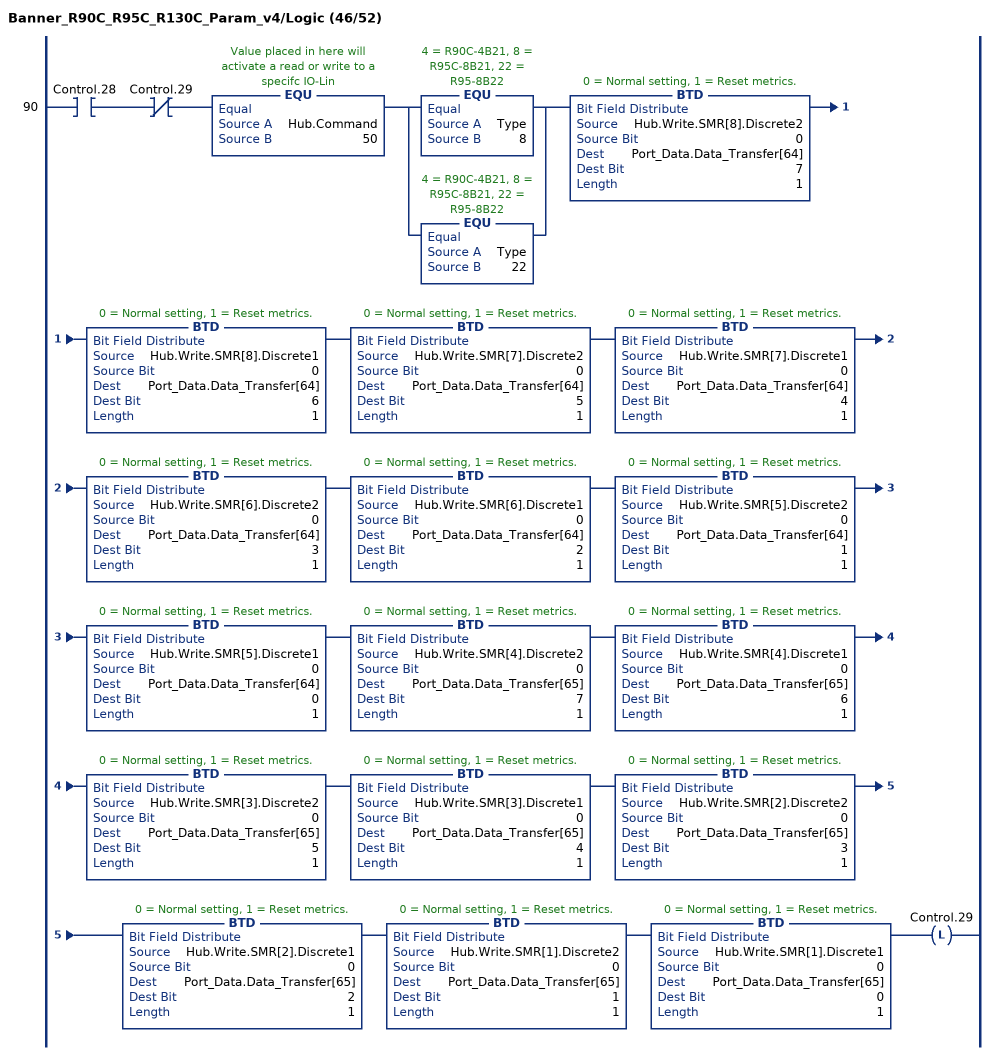
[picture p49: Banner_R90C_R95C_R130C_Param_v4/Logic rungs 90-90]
   90: XIC(Control.28)XIO(Control.29)EQU(Hub.Command,50)[EQU(Type,8) ,EQU(Type,22) ]BTD(Hub.Write.SMR[8].Discrete2,0,Port_Data.Data_Transfer[64],7,1)BTD(Hub.Write.SMR[8].Discrete1,0,Port_Data.Data_Transfer[64],6,1)BTD(Hub.Write.SMR[7].Discrete2,0,Port_Data.Data_Transfer[64],5,1)BTD(Hub.Write.SMR[7].Discrete1,0,Port_Data.Data_Transfer[64],4,1)BTD(Hub.Write.SMR[6].Discrete2,0,Port_Data.Data_Transfer[64],3,1)BTD(Hub.Write.SMR[6].Discrete1,0,Port_Data.Data_Transfer[64],2,1)BTD(Hub.Write.SMR[5].Discrete2,0,Port_Data.Data_Transfer[64],1,1)BTD(Hub.Write.SMR[5].Discrete1,0,Port_Data.Data_Transfer[64],0,1)BTD(Hub.Write.SMR[4].Discrete2,0,Port_Data.Data_Transfer[65],7,1)BTD(Hub.Write.SMR[4].Discrete1,0,Port_Data.Data_Transfer[65],6,1)BTD(Hub.Write.SMR[3].Discrete2,0,Port_Data.Data_Transfer[65],5,1)BTD(Hub.Write.SMR[3].Discrete1,0,Port_Data.Data_Transfer[65],4,1)BTD(Hub.Write.SMR[2].Discrete2,0,Port_Data.Data_Transfer[65],3,1)BTD(Hub.Write.SMR[2].Discrete1,0,Port_Data.Data_Transfer[65],2,1)BTD(Hub.Write.SMR[1].Discrete2,0,Port_Data.Data_Transfer[65],1,1)BTD(Hub.Write.SMR[1].Discrete1,0,Port_Data.Data_Transfer[65],0,1)OTL(Control.29);
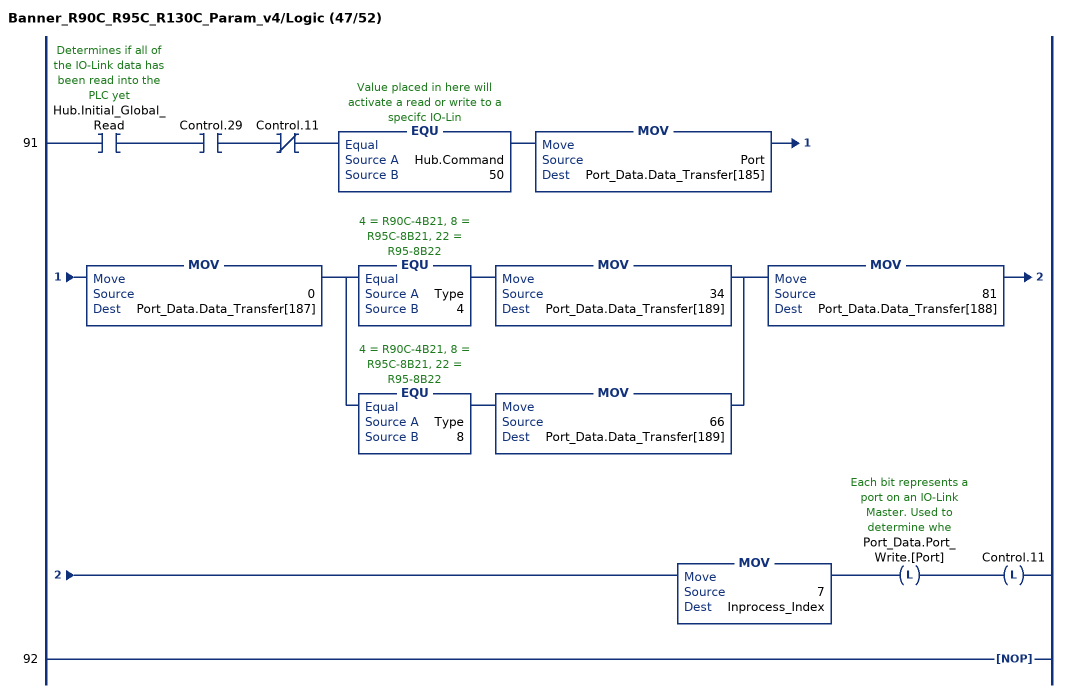
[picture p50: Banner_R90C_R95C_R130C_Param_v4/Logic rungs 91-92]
   91: XIC(Hub.Initial_Global_Read)XIC(Control.29)XIO(Control.11)EQU(Hub.Command,50)MOV(Port,Port_Data.Data_Transfer[185])MOV(0,Port_Data.Data_Transfer[187])[EQU(Type,4) MOV(34,Port_Data.Data_Transfer[189]) ,EQU(Type,8) MOV(66,Port_Data.Data_Transfer[189]) ]MOV(81,Port_Data.Data_Transfer[188])MOV(7,Inprocess_Index)OTL(Port_Data.Port_Write.[Port])OTL(Control.11);
   92: NOP();
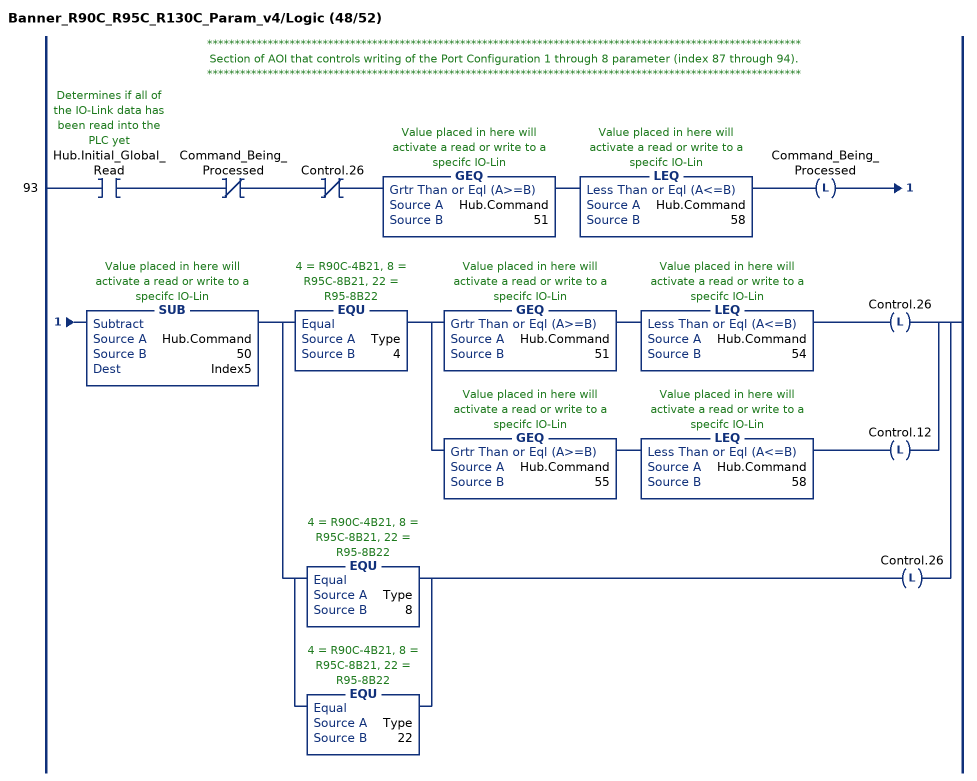
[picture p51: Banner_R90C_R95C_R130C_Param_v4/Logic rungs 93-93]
   // ************************************************************************************************************
   // Section of AOI that controls writing of the Port Configuration 1 through 8 parameter (index 87 through 94).
   // ************************************************************************************************************
   93: XIC(Hub.Initial_Global_Read)XIO(Command_Being_Processed)XIO(Control.26)GEQ(Hub.Command,51)LEQ(Hub.Command,58)OTL(Command_Being_Processed)SUB(Hub.Command,50,Index5)[EQU(Type,4) [GEQ(Hub.Command,51) LEQ(Hub.Command,54) OTL(Control.26) ,GEQ(Hub.Command,55) LEQ(Hub.Command,58) OTL(Control.12) ] ,[EQU(Type,8) ,EQU(Type,22) ] OTL(Control.26) ];
